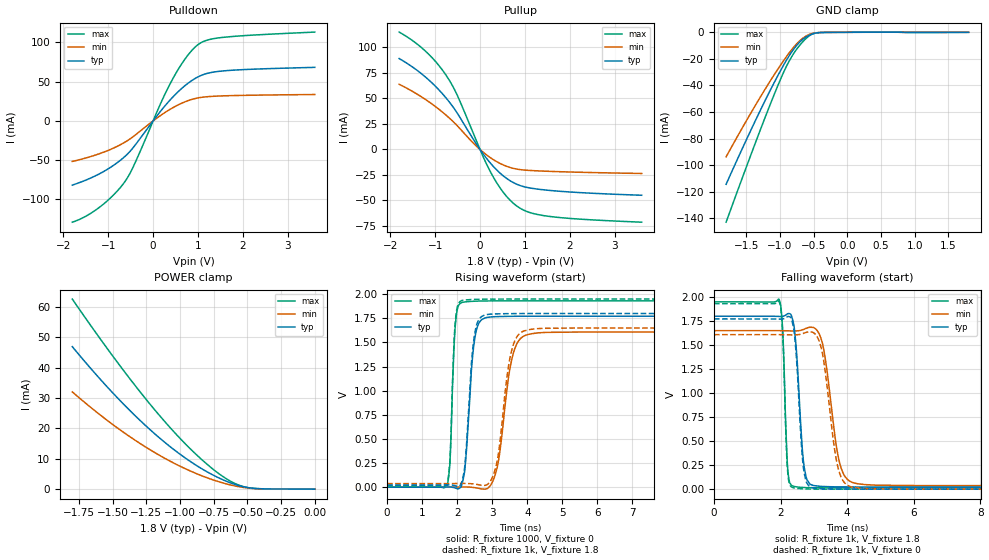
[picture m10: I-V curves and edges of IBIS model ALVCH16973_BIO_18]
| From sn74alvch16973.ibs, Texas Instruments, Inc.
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[Model]   ALVCH16973_BIO_18
Model_type  I/O
Vinl=0.5775
Vinh=1.2675
Enable   Active-Low
Vref =   0
Rref =   1000
Cref =   30p
Vmeas =   0.9
| variable   typ   min   max
C_comp   3.26pF   2.95pF   3.48pF
| C_pullup   4.49pF   3.43pF   4.99pF
| C_pulldown   4.82pF   3.15pF   6.41pF
| C_tri-state   3.26pF   2.95pF   3.48pF
[Temperature Range]   40   100   -40
| Ambient temperature   25   85   -40
[Voltage range]   1.8   1.65   1.95
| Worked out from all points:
|   slope of the pulldown table from 0 to 0.27 V, typ, clamps not added: 13.8 ohm
|   slope of the pullup table from 0 to 0.27 V, typ, clamps not added: 17.6 ohm
|   GND clamp passes 1 mA (typ) near -0.50 V on its own axis
|   POWER clamp passes 1 mA (typ) near -0.55 V on its own axis
|   rising waveform, R_fixture 1000, V_fixture 0: 20-80 % time 199ps typ, 337ps min, 113ps max; typ from 0 V to 1.77 V
|   falling waveform, R_fixture 1k, V_fixture 1.8: 20-80 % time 188ps typ, 365ps min, 109ps max; typ from 1.8 V to 0.023 V
|   rising waveform, R_fixture 1k, V_fixture 1.8: 20-80 % time 193ps typ, 318ps min, 110ps max; typ from 0.023 V to 1.8 V
|   falling waveform, R_fixture 1k, V_fixture 0: 20-80 % time 183ps typ, 349ps min, 107ps max; typ from 1.77 V to 0 V
[GND Clamp]
| ALVCH16973_BIO_18
|   Voltage   I(typ)   I(min)   I(max)
-1.8V     -114.4mA   -93.74mA   -142.9mA
-1.55V    -86.48mA   -71.1mA    -108.3mA
-1.325V   -62.23mA   -51.54mA   -77.86mA
-1.12V    -41.21mA   -34.65mA   -51.11mA
-965mV    -26.41mA   -22.72mA   -32.22mA
-875mV    -18.58mA   -16.31mA   -22.75mA
-785mV    -11.9mA    -10.53mA   -15.06mA
-680mV    -6.088mA   -5.234mA   -8.189mA
-580mV    -2.563mA   -1.963mA   -3.232mA
-495mV    -862.4uA   -609.1uA   -886.9uA
-380mV    -137.5uA   -100.9uA   -157.2uA
1.8V      633.6pA    17.14uA    -35.19uA
[POWER Clamp]
| ALVCH16973_BIO_18
|   Voltage   I(typ)   I(min)   I(max)
-1.8V     46.9mA     32mA       62.55mA
-1.505V   31.94mA    21.45mA    44.13mA
-1.37V    25.77mA    17.18mA    36.18mA
-1.235V   20.07mA    13.3mA     28.63mA
-1.1V     14.92mA    9.837mA    21.56mA
-975mV    10.69mA    7.019mA    15.55mA
-860mV    7.289mA    4.782mA    10.58mA
-745mV    4.421mA    2.907mA    6.209mA
-615mV    1.894mA    1.281mA    2.37mA
-500mV    537.7uA    395.3uA    541.3uA
-375mV    99.26uA    77.48uA    115.9uA
-16.28fV  633.6pA    1.888nA    58.65pA
[Pulldown]
| ALVCH16973_BIO_18
|   Voltage   I(typ)   I(min)   I(max)
-1.8V     -81.77mA   -51.62mA   -129mA
-1.175V   -66.78mA   -41.36mA   -109.2mA
-875mV    -56.33mA   -34.41mA   -93.93mA
-630mV    -45.37mA   -27.16mA   -77.47mA
-430mV    -33mA      -19.38mA   -56.92mA
150mV     11.21mA    6.297mA    20.03mA
405mV     28.31mA    15.69mA    50.14mA
710mV     44.96mA    24.35mA    78.83mA
990mV     55.79mA    29.2mA     96.74mA
1.2V      60.49mA    30.8mA     102.8mA
1.555V    63.68mA    31.91mA    106.4mA
3.6V      68.24mA    33.63mA    113.2mA
[Pullup]
| ALVCH16973_BIO_18
|   Voltage   I(typ)   I(min)   I(max)
-1.8V     89.09mA    63.89mA    115mA
-1.22V    71.17mA    49.14mA    96.57mA
-975mV    61.12mA    41.42mA    85.41mA
-755mV    50.4mA     33.55mA    72.69mA
-505mV    35.45mA    23.15mA    52.97mA
-50mV     3.259mA    2.011mA    5.287mA
245mV     -14.09mA   -8.478mA   -22.97mA
515mV     -25.78mA   -15.14mA   -41.86mA
790mV     -33.53mA   -19.02mA   -54.5mA
1.08V     -37.51mA   -20.51mA   -61.41mA
1.505V    -39.97mA   -21.4mA    -65.42mA
3.6V      -44.91mA   -23.56mA   -71.31mA
[Ramp]
| ALVCH16973_BIO_18
| variable   typ   min   max
dV/dt_r   1.07/2.17E-10   0.98/3.50E-10   1.16/1.21E-10
dV/dt_f   1.08/2.04E-10   0.99/3.79E-10   1.18/1.13E-10
R_load = 1000
[Rising Waveform]
| ALVCH16973_BIO_18
R_fixture =   1000
C_fixture =   0
L_fixture =   0
V_fixture =   0
V_fixture_min = 0
V_fixture_max = 0
|   Time   V(typ)   V(min)   V(max)
0s        5.832nV    32.59nV    120.7pV
1.72ns    1.377mV    -47.76uV   16.94mV
1.95ns    -8.982mV   479.6uV    1.688V
2.19ns    114.3mV    1.994mV    1.919V
2.49ns    1.51V      -4.125mV   1.928V
2.875ns   1.761V     -10.15mV   1.931V
3.16ns    1.768V     235.2mV    1.931V
3.605ns   1.771V     1.393V     1.931V
4.135ns   1.772V     1.591V     1.932V
29.99ns   1.772V     1.608V     1.932V
[Falling Waveform]
| ALVCH16973_BIO_18
R_fixture =   1k
C_fixture =   0
L_fixture =   0
V_fixture =   1.8
V_fixture_min = 1.65
V_fixture_max = 1.95
|   Time   V(typ)   V(min)   V(max)
0s        1.8V       1.65V      1.95V
1.96ns    1.798V     1.65V      1.97V
2.065ns   1.8V       1.649V     1.646V
2.22ns    1.827V     1.648V     189.6mV
2.465ns   1.49V      1.647V     24.54mV
2.795ns   96.85mV    1.677V     15.98mV
3.255ns   28.48mV    1.522V     14.24mV
3.815ns   23.64mV    222.2mV    13.98mV
4.315ns   23.14mV    56.14mV    13.96mV
29.99ns   23.03mV    37.16mV    13.95mV
[Rising Waveform]
| ALVCH16973_BIO_18
R_fixture =   1k
C_fixture =   0
L_fixture =   0
V_fixture =   1.8
V_fixture_min = 1.65
V_fixture_max = 1.95
|   Time   V(typ)   V(min)   V(max)
0s        23.03mV    37.16mV    13.95mV
1.72ns    24.28mV    37.14mV    32.32mV
1.945ns   14.6mV     37.61mV    1.705V
2.18ns    126.4mV    38.8mV     1.939V
2.485ns   1.554V     32.56mV    1.946V
2.87ns    1.791V     29.99mV    1.949V
3.15ns    1.797V     286mV      1.95V
3.575ns   1.799V     1.446V     1.95V
4.09ns    1.8V       1.635V     1.95V
29.99ns   1.8V       1.65V      1.95V
[Falling Waveform]
| ALVCH16973_BIO_18
R_fixture =   1k
C_fixture =   0
L_fixture =   0
V_fixture =   0
V_fixture_min = 0
V_fixture_max = 0
|   Time   V(typ)   V(min)   V(max)
0s        1.772V     1.608V     1.932V
1.96ns    1.77V      1.608V     1.95V
2.065ns   1.772V     1.608V     1.608V
2.21ns    1.797V     1.607V     193.5mV
2.425ns   1.584V     1.606V     11.49mV
2.685ns   228.9mV    1.621V     3.341mV
2.985ns   11.87mV    1.63V      755.3uV
3.73ns    642.9uV    217mV      38.35uV
4.215ns   105.5uV    16.41mV    5.729uV
29.99ns   15.78nV    46.62nV    3.786nV
